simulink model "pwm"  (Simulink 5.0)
settings: Solver=ode45  StartTime=9.000000000000001E-004  StopTime=9.500000000000001E-004  FixedStep=0.000001  RelTol=1e-3

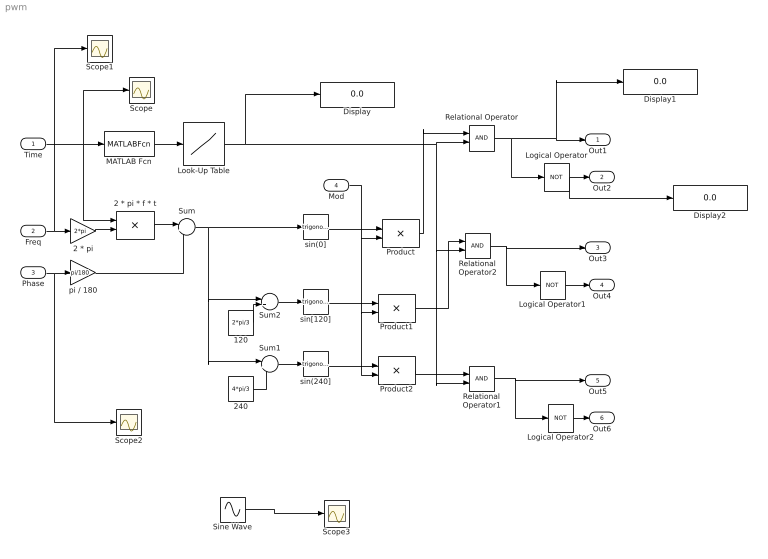
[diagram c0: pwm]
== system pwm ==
  Time : Inport
  Freq : Inport  Port=2
  Phase : Inport  Port=3
  Mod : Inport  Port=4
  120 : Constant  Value=2*pi/3
  2 * pi : Gain  Gain=2*pi
  2 * pi * f * t : Product
  240 : Constant  Value=4*pi/3
  Display : Display
  Display1 : Display
  Display2 : Display
  Logical Operator : Logic  Operator=NOT
  Logical Operator1 : Logic  Operator=NOT
  Logical Operator2 : Logic  Operator=NOT
  Look-Up Table : Lookup  InputValues=[0 1/(4*2000) 3/(4*2000) 1/2000]  OutputValues=[0 1 -1 0]
  MATLAB Fcn : MATLABFcn  MATLABFcn=mod( u, 1/2000)
  Product : Product
  Product1 : Product
  Product2 : Product
  Relational Operator : RelationalOperator
  Relational Operator1 : RelationalOperator
  Relational Operator2 : RelationalOperator
  Scope{,1..3} (4 alike) : Scope
  Sine Wave : Sin  Frequency=50  SampleTime=0  VectorParams1D=off
  Sum : Sum  Inputs=|++
  Sum1 : Sum  Inputs=|++
  Sum2 : Sum  Inputs=|++
  pi / 180 : Gain  Gain=pi/180
  sin(0] : Trigonometry
  sin(240] : Trigonometry
  sin[120] : Trigonometry
  Out1 : Outport
  Out2 : Outport  Port=2
  Out3 : Outport  Port=3
  Out4 : Outport  Port=4
  Out5 : Outport  Port=5
  Out6 : Outport  Port=6
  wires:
  MATLAB Fcn/1 -> Look-Up Table/1
  Time/1 -> MATLAB Fcn/1, 2 * pi * f * t/1, Scope/1
  sin[120]/1 -> Product1/1
  sin(0]/1 -> Product/1
  sin(240]/1 -> Product2/1
  Sum1/1 -> sin(240]/1
  Freq/1 -> 2 * pi/1, Scope1/1
  2 * pi/1 -> 2 * pi * f * t/2
  Phase/1 -> Scope2/1, pi / 180/1
  2 * pi * f * t/1 -> Sum/1
  pi / 180/1 -> Sum/2
  Sum/1 -> sin(0]/1, Sum2/1, Sum1/1
  Sum2/1 -> sin[120]/1
  Mod/1 -> Product/2, Product1/2, Product2/2
  120/1 -> Sum2/2
  240/1 -> Sum1/2
  Product/1 -> Relational Operator/1
  Product1/1 -> Relational Operator2/1
  Product2/1 -> Relational Operator1/1
  Relational Operator/1 -> Logical Operator/1, Out1/1, Display1/1
  Relational Operator2/1 -> Out3/1, Logical Operator1/1
  Logical Operator1/1 -> Out4/1
  Relational Operator1/1 -> Out5/1, Logical Operator2/1
  Logical Operator2/1 -> Out6/1
  Look-Up Table/1 -> Relational Operator/2, Relational Operator2/2, Relational Operator1/2, Display/1
  Logical Operator/1 -> Out2/1, Display2/1
  Sine Wave/1 -> Scope3/1
